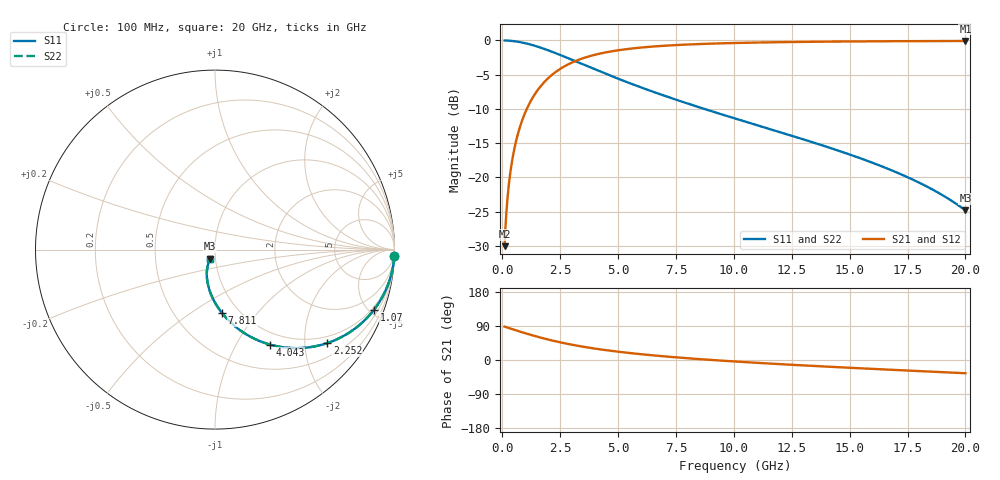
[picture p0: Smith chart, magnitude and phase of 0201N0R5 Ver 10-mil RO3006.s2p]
# GHz S MA R 50
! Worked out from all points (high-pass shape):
!   1601 points, 100 MHz to 20 GHz, reference 50 ohm
!   highest |S21| = -0.08 dB at 20 GHz (marker M1); lowest = -30.1 dB at 100 MHz (marker M2)
!   |S21| within 3 dB of the highest: 3.111 GHz to end of sweep
!   lowest |S11| = -24.8 dB at 20 GHz (marker M3), VSWR 1.12, Z = 47.2 - j4.8 ohm
!   |S11| at or under -10 dB: 8.721 GHz to end of sweep
!   |S22| runs from -24.8 to 0.0 dB; largest |S21 - S12| = 0
!   S11 on the Smith chart (normalised r, x): 100 MHz: 1, -57; 1.07 GHz: 0.82, -5.35; 2.252 GHz: 0.82, -2.53; 4.043 GHz: 0.82, -1.39; 7.811 GHz: 0.83, -0.67; 20 GHz: 0.94, -0.10
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0.1  0.9995 -2.0  0.03144 88.0  0.03144 88.0  0.9995 -2.0
0.14975  0.9989 -3.0  0.04705 87.0  0.04705 87.0  0.9989 -3.0
0.2368125  0.9972 -4.7  0.07428 85.3  0.07428 85.3  0.9972 -4.7
0.2865625  0.9959 -5.7  0.08977 84.3  0.08977 84.3  0.9959 -5.7
0.3611875  0.9936 -7.2  0.1129 82.8  0.1129 82.8  0.9936 -7.2
0.4606875  0.9896 -9.2  0.1434 80.8  0.1434 80.8  0.9896 -9.2
0.5850625  0.9834 -11.6  0.181 78.4  0.181 78.4  0.9834 -11.6
0.721875  0.975 -14.2  0.2215 75.8  0.2215 75.8  0.975 -14.2
1.070125  0.9474 -20.7  0.3192 69.2  0.3192 69.2  0.9474 -20.7
1.5925  0.8931 -29.8  0.4484 60.1  0.4484 60.1  0.8931 -29.8
2.251688  0.8139 -39.8  0.5791 50.1  0.5791 50.1  0.8139 -39.8
2.7865  0.7485 -46.8  0.6608 43.0  0.6608 43.0  0.7485 -46.8
3.420812  0.6753 -54.0  0.7348 35.8  0.7348 35.8  0.6753 -54.0
4.042688  0.6106 -60.0  0.7888 29.7  0.7888 29.7  0.6106 -60.0
5.274  0.5042 -69.7  0.8599 19.9  0.8599 19.9  0.5042 -69.7
6.741625  0.4087 -78.5  0.9085 10.9  0.9085 10.9  0.4087 -78.5
7.81125  0.3547 -83.8  0.9304 5.5  0.9304 5.5  0.3547 -83.8
10.05  0.2691 -92.9  0.9579 -4.0  0.9579 -4.0  0.2691 -92.9
13.37081  0.1811 -103.7  0.9775 -15.5  0.9775 -15.5  0.1811 -103.7
16.69162  0.1148 -112.3  0.9866 -25.5  0.9866 -25.5  0.1148 -112.3
18.48262  0.08317 -116.0  0.9894 -30.7  0.9894 -30.7  0.08317 -116.0
20  0.05743 -117.8  0.9908 -34.9  0.9908 -34.9  0.05743 -117.8
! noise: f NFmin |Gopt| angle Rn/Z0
0.1  0.00118  0.9727  1.148  0.009797
2.301  0.005395  0.8296  5.921  0.006651
4.515  0.008303  0.7862  10.01  0.007928
6.729  0.01081  0.7592  14.16  0.00896
8.943  0.01311  0.7398  18.3  0.009845
11.14  0.01526  0.7252  22.4  0.01063
13.36  0.01734  0.7137  26.49  0.01134
15.57  0.01935  0.7048  30.52  0.012
17.79  0.02132  0.6978  34.49  0.01262
20  0.02327  0.6925  38.4  0.01321
